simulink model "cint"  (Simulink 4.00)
settings: Solver=ode45  StartTime=0.0  StopTime=10.0  MaxStep=0.1  RelTol=1e-3  AbsTol=0.001
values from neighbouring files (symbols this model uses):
  A = [-1 2;-5 -3]    [cond_cint.m]    (also in EXAMPLE3.M = [Ao Bo*Cd; zeros(1,3) Ad]; EXAMPLE2.M = [Ao Bo*Cd; zeros(1,2) Ad]; EXAMPLE1.M = conv([1 -2],[1 0 36 0]))
  B = [-1 0;-1 2]    [cond_cint.m]    (also in EXAMPLE3.M = [Bo; 0]; EXAMPLE2.M = [Bo; 0]; EXAMPLE1.M = 1)
  C = [-1 0;1 1]    [cond_cint.m]    (also in EXAMPLE3.M = Cont_bi; [t,x,y1,y2,y3] = sim('closed_loop',5); EXAMPLE1.M = zpk(tf(conv(P',[1 9]),conv(conv(L',[1 3]),[1 0 36 0]))); EXAMPLE2.M = minreal( (tf(P',E)+series(Q,tf(Ao,E)))/(tf(L',E)-series(Q,tf)
  J = [-4 6;5 2]    [cond_cint.m]    (also in EXAMPLE3.M = (place(A', C', [-3 -4 -5 -6]))'; EXAMPLE2.M = (place(A', C', [-0.5 -0.7 -1]))')
  K = [-4.7065 -2.02 -8.0631 .0619; -4.8306 .3421 -8.0217 -4.0244]    [cond_cint.m]    (also in EXAMPLE3.M = [Ko Cd]; PAQ.M = P*fii; EXAMPLE2.M = [Ko Cd])

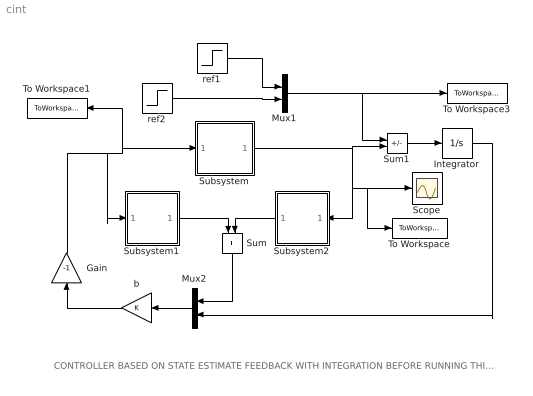
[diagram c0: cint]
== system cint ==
  note: CONTROLLER BASED ON STATE ESTIMATE FEEDBACK WITH INTEGRATION BEFORE RUNNING THIS SIMULATION, THE USER MUST ASSIGN VALUES TO THE PLANT STATE SPACE MATRICES A,B,C AND TO THE OBSERVER AND STATE GAINS J AND K, RESPECTIVELY. RUN M-FILE COND_CINT
  Gain : Gain  Orientation=up  Gain=-1  Multiplication=Element-wise(K.*u)  SaturateOnIntegerOverflow=on
  Integrator : Integrator  ExternalReset=none  InitialConditionSource=internal  InitialCondition=0  LimitOutput=off  UpperSaturationLimit=inf  LowerSaturationLimit=-inf  ShowSaturationPort=off  ShowStatePort=off  AbsoluteTolerance=auto
  Mux1 : Mux  Inputs=2
  Mux2 : Mux  Orientation=left  Inputs=2
  Scope : Scope
  Subsystem : Subsystem  mask{A=A, B=B, C=C}
  Subsystem1 : Subsystem  mask{A=A, B=B, C=C, J=J}
      mask init:
      | AT1=A-J*C; CT1=eye(size(A)); BT1=B;
  Subsystem2 : Subsystem  Orientation=left  mask{A=A, C=C, J=J}
      mask init:
      | AT2=A-J*C;BT2=J;CT2=eye(size(A));
  Sum : Sum  Orientation=down  Inputs=++
  Sum1 : Sum  Inputs=+-
  To Workspace : ToWorkspace  VariableName=y  SampleTime=-1  SaveFormat=Array
  To Workspace1 : ToWorkspace  VariableName=u  SampleTime=-1  SaveFormat=Array
  To Workspace3 : ToWorkspace  VariableName=r  SampleTime=-1  SaveFormat=Array
  b : Gain  Orientation=left  Gain=K  Multiplication=Matrix(K*u)  SaturateOnIntegerOverflow=on
  ref1 : Step  Time=0  Before=0  After=1  SampleTime=0
  ref2 : Step  Time=5  Before=0  After=-1  SampleTime=0
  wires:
  Subsystem/1(Out1) -> Sum1/2, Scope/1, To Workspace/1, Subsystem2/1(In1)
  Subsystem1/1(Out1) -> Sum/1
  Subsystem2/1(Out1) -> Sum/2
  Sum1/1 -> Integrator/1
  Sum/1 -> Mux2/1
  Integrator/1 -> Mux2/2
  Mux2/1 -> b/1
  ref2/1 -> Mux1/2
  Mux1/1 -> Sum1/1, To Workspace3/1
  ref1/1 -> Mux1/1
  b/1 -> Gain/1
  Gain/1 -> Subsystem1/1(In1), Subsystem/1(In1), To Workspace1/1

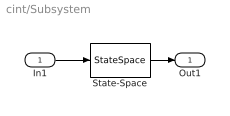
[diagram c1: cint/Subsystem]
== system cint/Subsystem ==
  In1 : Inport  Port=1  LatchInput=off
  State-Space : StateSpace  A=A  B=B  C=C  D=0*C*B  X0=0  AbsoluteTolerance=auto  Realization=auto
  Out1 : Outport  Port=1
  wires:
  In1/1 -> State-Space/1
  State-Space/1 -> Out1/1

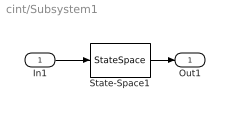
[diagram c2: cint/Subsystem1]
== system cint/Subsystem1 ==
  In1 : Inport  Port=1  LatchInput=off
  State-Space1 : StateSpace  A=AT1  B=BT1  C=CT1  D=0*BT1  X0=0  AbsoluteTolerance=auto  Realization=auto
  Out1 : Outport  Port=1
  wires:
  In1/1 -> State-Space1/1
  State-Space1/1 -> Out1/1

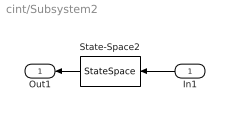
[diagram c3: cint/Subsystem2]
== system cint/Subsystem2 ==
  In1 : Inport  Orientation=left  Port=1  LatchInput=off
  State-Space2 : StateSpace  Orientation=left  A=AT2  B=BT2  C=CT2  D=0* BT2  X0=0  AbsoluteTolerance=auto  Realization=auto
  Out1 : Outport  Orientation=left  Port=1
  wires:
  In1/1 -> State-Space2/1
  State-Space2/1 -> Out1/1
